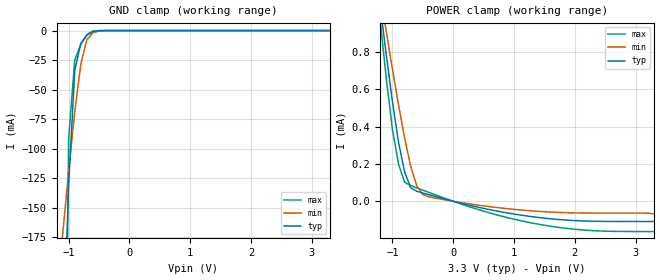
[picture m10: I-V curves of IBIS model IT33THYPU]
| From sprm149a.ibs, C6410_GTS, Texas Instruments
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[Model]   IT33THYPU
Model_type   Input
Polarity   Non-Inverting
| signals   A, Y
Vinl = 0.8V
Vinh = 2.0V
|   typ   min   max
C_comp   1.5797p   1.5046p   1.7659p
|   typ   min   max
[Temperature Range]   25   -40   125
|   typ   min   max
[Voltage Range]   3.30V   3.00V   3.60V
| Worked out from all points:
|   GND clamp passes 1 mA (typ) near -0.61 V on its own axis
|   POWER clamp passes 1 mA (typ) near -1.18 V on its own axis
[GND_clamp]
|   Voltage   I(typ)   I(min)   I(max)
-3.3V     -4.395A    -1.514A    -19.03A
-1.1V     -280.5mA   -173.1mA   -561.2mA
-1V       -130.2mA   -118.7mA   -91.18mA
-900mV    -33.58mA   -68.65mA   -24.89mA
-800mV    -10.81mA   -28.33mA   -11.69mA
-700mV    -3.883mA   -7.526mA   -3.315mA
-600mV    -741.7uA   -1.835mA   -366.6uA
-500mV    -67.31uA   -328.9uA   -17.03uA
-400mV    -3.756uA   -40.45uA   -379.9nA
3.3V      222pA      34.37nA    133.2pA
[POWER_clamp]
|   Voltage   I(typ)   I(min)   I(max)
-3.3V     6.878mA    5.575mA    8.077mA
-1.2V     1.04mA     1.107mA    962.3uA
-1.1V     780.5uA    904.7uA    653.7uA
-1V       533.3uA    707uA      383.6uA
-900mV    316uA      516.3uA    199uA
-800mV    157.4uA    338.5uA    102.4uA
-700mV    72.96uA    187.6uA    83.65uA
-600mV    53.67uA    82.48uA    71.5uA
-500mV    44.14uA    35.96uA    59.41uA
500mV     -38.05uA   -24.41uA   -52.82uA
1.4V      -86.48uA   -53.81uA   -122.5uA
3.3V      -108.4uA   -67.2uA    -162.2uA
